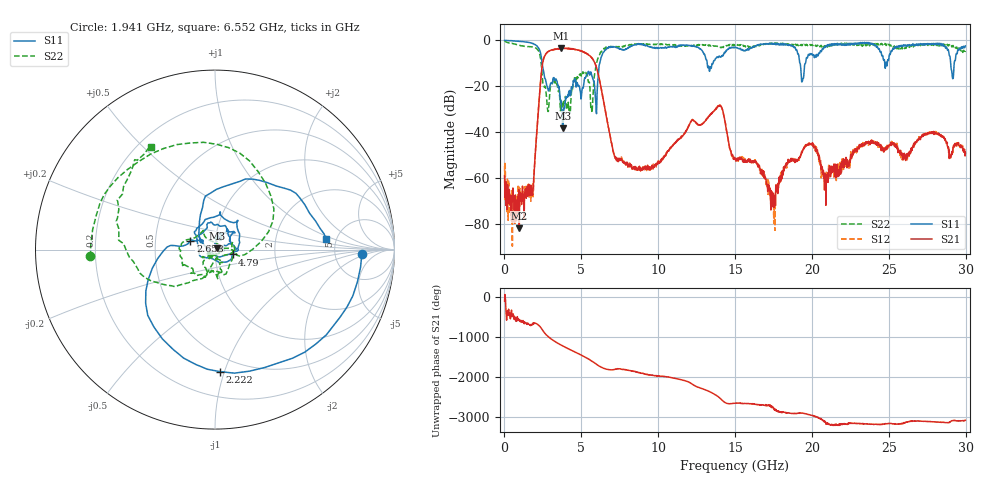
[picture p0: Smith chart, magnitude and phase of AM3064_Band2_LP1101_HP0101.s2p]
# Hz S DB R 50.0
!freq dBS11 angS11 dBS21 angS21 dBS12 angS12 dBS22 angS22
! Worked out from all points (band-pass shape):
!   1600 points, 10 MHz to 29.98 GHz, reference 50 ohm
!   highest |S21| = -3.37 dB at 3.703 GHz (marker M1); lowest = -81.7 dB at 965.9 MHz (marker M2)
!   |S21| within 3 dB of the highest: 2.65 GHz to 5.48 GHz (2.831 GHz wide, 69.6 % of centre)
!   lowest |S11| = -38.3 dB at 3.796 GHz (marker M3), VSWR 1.02, Z = 51.1 + j0.629 ohm
!   |S11| at or under -10 dB: 2.45 GHz to 6.198 GHz (3.747 GHz wide, 86.7 % of centre); 13.19 GHz to 13.57 GHz (378.6 MHz wide, 2.83 % of centre); 19.23 GHz to 19.57 GHz (348.5 MHz wide, 1.8 % of centre)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
!   |S22| runs from -32.0 to -0.2 dB; largest |S21 - S12| = 0.02
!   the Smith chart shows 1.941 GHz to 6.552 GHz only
!   S11 on the Smith chart (normalised r, x): 1.941 GHz: 9.84, -1.34; 2.222 GHz: 0.38, -0.97; 2.653 GHz: 0.75, +0.08; 4.79 GHz: 1.22, -0.07; 6.552 GHz: 4.12, +0.77
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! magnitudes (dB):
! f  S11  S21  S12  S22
! 10 MHz  0.0  -59.0  -54.6  -0.2
! 965.9 MHz  -0.4  -81.7  -68.8  -2.1
! 1.941 GHz  -1.7  -56.0  -56.0  -3.2
! 2.222 GHz  -3.3  -29.0  -28.8  -4.6
! 2.653 GHz  -16.7  -6.3  -6.3  -20.0
! 3.703 GHz  -28.0  -3.4  -3.5  -27.0
! 3.796 GHz  -38.3  -3.5  -3.4  -29.7
! 4.79 GHz  -19.9  -4.3  -4.2  -16.1
! 5.015 GHz  -23.7  -4.7  -4.7  -15.8
! 5.671 GHz  -15.2  -7.5  -7.5  -29.8
! 5.952 GHz  -28.1  -11.1  -11.1  -11.0
! 6.552 GHz  -4.1  -30.4  -30.3  -3.4
! 7.301 GHz  -3.1  -52.3  -51.7  -2.7
! 10 GHz  -3.4  -52.8  -53.1  -1.8
! 13.97 GHz  -7.0  -28.6  -28.3  -2.8
! 15 GHz  -2.9  -51.7  -51.8  -1.9
! 17.46 GHz  -1.3  -72.1  -68.9  -1.3
! 19.37 GHz  -17.8  -48.4  -48.6  -2.0
! 19.99 GHz  -5.8  -45.3  -45.3  -1.9
! 20.93 GHz  -2.4  -58.7  -58.0  -2.2
! 25 GHz  -8.1  -45.8  -46.0  -1.7
! 29.98 GHz  -2.4  -49.2  -49.4  -4.6
